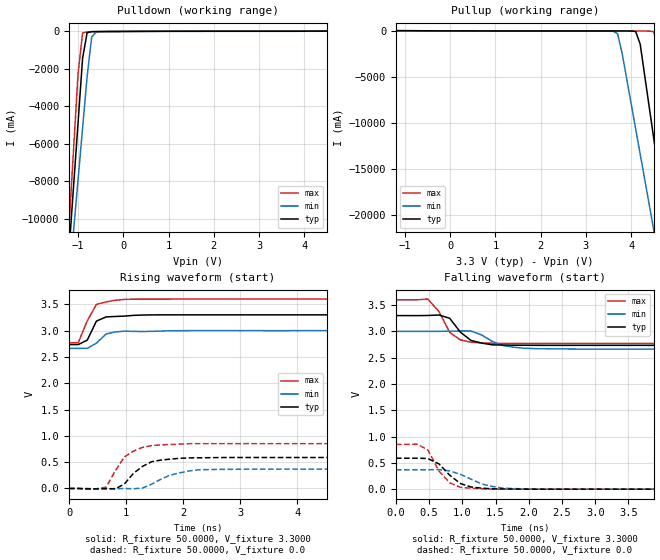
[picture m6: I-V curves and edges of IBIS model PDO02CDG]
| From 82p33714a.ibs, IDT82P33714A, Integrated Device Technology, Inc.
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|   Model PDO02CDG
[Model]  PDO02CDG
Model_type Output
Polarity   Non-Inverting
Vmeas =  1.6500V
Cref =   50.0000pF
Rref =   1.0000M
Vref =   0.0V
C_comp   70.2000fF   57.9000fF   75.6000fF
[Temperature Range]   25.0000   0.1250k   -40.0000
[Voltage Range]   3.3000V   3.0000V   3.6000V
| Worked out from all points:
|   slope of the pulldown table from 0 to 0.495 V, typ, clamps not added: 93.5 ohm
|   slope of the pullup table from 0 to 0.495 V, typ, clamps not added: 103 ohm
|   rising waveform, R_fixture 50.0000, V_fixture 3.3000: 20-80 % time 160ps typ, 217ps min, 223ps max; typ from 2.73 V to 3.3 V
|   rising waveform, R_fixture 50.0000, V_fixture 0.0: 20-80 % time 384ps typ, 503ps min, 363ps max; typ from 0 V to 0.588 V
|   falling waveform, R_fixture 50.0000, V_fixture 3.3000: 20-80 % time 262ps typ, 328ps min, 254ps max; typ from 3.3 V to 2.73 V
|   falling waveform, R_fixture 50.0000, V_fixture 0.0: 20-80 % time 304ps typ, 438ps min, 266ps max; typ from 0.588 V to 0 V
[Pulldown]
|Voltage   I(typ)   I(min)   I(max)
-3.3V     -83.46A    -71.04A    -95.7A
-1.2V     -11.69A    -13.39A    -10.37A
-1.1V     -8.277A    -10.65A    -6.308A
-1V       -4.856A    -7.901A    -2.242A
-900mV    -1.434A    -5.152A    -75.7mA
-800mV    -65.16mA   -2.403A    -21.08mA
-700mV    -11.27mA   -303.5mA   -14.04mA
-600mV    -7.391mA   -27.24mA   -9.673mA
6.6V      40.22mA    13.56mA    62.13mA
[Pullup]
|Voltage   I(typ)   I(min)   I(max)
-3.3V     28.25mA    4.656mA    56.59mA
3.6V      -12.04mA   -30.45mA   -17.4mA
3.7V      -12.06mA   -307.3mA   -17.43mA
3.8V      -12.11mA   -2.408A    -17.46mA
4.1V      -69.23mA   -10.65A    -17.6mA
4.2V      -1.441A    -13.4A     -18.36mA
4.5V      -11.7A     -21.65A    -82.29mA
4.6V      -15.13A    -24.39A    -2.253A
4.8V      -21.97A    -29.89A    -10.38A
5V        -28.81A    -35.38A    -18.52A
5.1V      -32.23A    -38.13A    -22.59A
6.6V      -83.47A    -79.27A    -83.54A
[Ramp]
| variable   typ   min   max
dV/dt_r  0.3530/0.3844n   0.2212/0.4930n   0.5110/0.3630n
dV/dt_f  0.3396/0.2623n   0.2022/0.3186n   0.4986/0.2510n
R_load = 50.0000
[Rising Waveform]
R_fixture= 50.0000
V_fixture= 3.3000
V_fixture_min= 3.0000
V_fixture_max= 3.6000
L_fixture= 0.0H
C_fixture= 0.0F
|time   V(typ)   V(min)   V(max)
0s        2.734V     2.663V     2.769V
160ps     2.734V     2.663V     2.768V
320ps     2.82V      2.662V     3.188V
480ps     3.181V     2.762V     3.499V
650ps     3.261V     2.936V     3.546V
810ps     3.269V     2.975V     3.578V
970ps     3.276V     2.99V      3.593V
1.29ns    3.296V     2.983V     3.599V
1.62ns    3.3V       2.992V     3.599V
16ns      3.3V       3V         3.6V
[Rising Waveform]
R_fixture= 50.0000
V_fixture= 0.0
V_fixture_min= 0.0
V_fixture_max= 0.0
L_fixture= 0.0H
C_fixture= 0.0F
|time   V(typ)   V(min)   V(max)
0s        7.011uV    7.347uV    6.889uV
650ps     -2.872mV   -5.444mV   22.73mV
810ps     -8.827mV   -2.518mV   335mV
970ps     85.13mV    -1.489mV   599.3mV
1.13ns    288.1mV    -5.225mV   709.9mV
1.29ns    421.3mV    8.099mV    782.5mV
1.62ns    541.9mV    182.4mV    828.5mV
2.1ns     581mV      332.4mV    850.5mV
2.59ns    586.5mV    361.9mV    851.3mV
16ns      588.4mV    368.7mV    851.6mV
[Falling Waveform]
R_fixture= 50.0000
V_fixture= 3.3000
V_fixture_min= 3.0000
V_fixture_max= 3.6000
L_fixture= 0.0H
C_fixture= 0.0F
|time   V(typ)   V(min)   V(max)
0s        3.3V       3V         3.6V
480ps     3.302V     2.999V     3.614V
650ps     3.311V     3V         3.372V
810ps     3.248V     3.004V     2.98V
970ps     2.985V     3.007V     2.837V
1.13ns    2.827V     3.007V     2.794V
1.45ns    2.744V     2.809V     2.773V
1.78ns    2.737V     2.698V     2.77V
2.59ns    2.734V     2.665V     2.769V
16ns      2.734V     2.663V     2.769V
[Falling Waveform]
R_fixture= 50.0000
V_fixture= 0.0
V_fixture_min= 0.0
V_fixture_max= 0.0
L_fixture= 0.0H
C_fixture= 0.0F
|time   V(typ)   V(min)   V(max)
0s        588.4mV    368.7mV    851.7mV
320ps     588.8mV    368.6mV    854.8mV
480ps     582.9mV    368.8mV    746.5mV
650ps     478.5mV    371.4mV    342.9mV
810ps     265mV      346.2mV    119.4mV
970ps     107.2mV    282.7mV    35.4mV
1.29ns    19.2mV     99.9mV     8.654mV
1.62ns    3.531mV    18.39mV    397.3uV
2.26ns    -68.32uV   501uV      90.27uV
16ns      -5.202uV   -6.911uV   12.03uV
